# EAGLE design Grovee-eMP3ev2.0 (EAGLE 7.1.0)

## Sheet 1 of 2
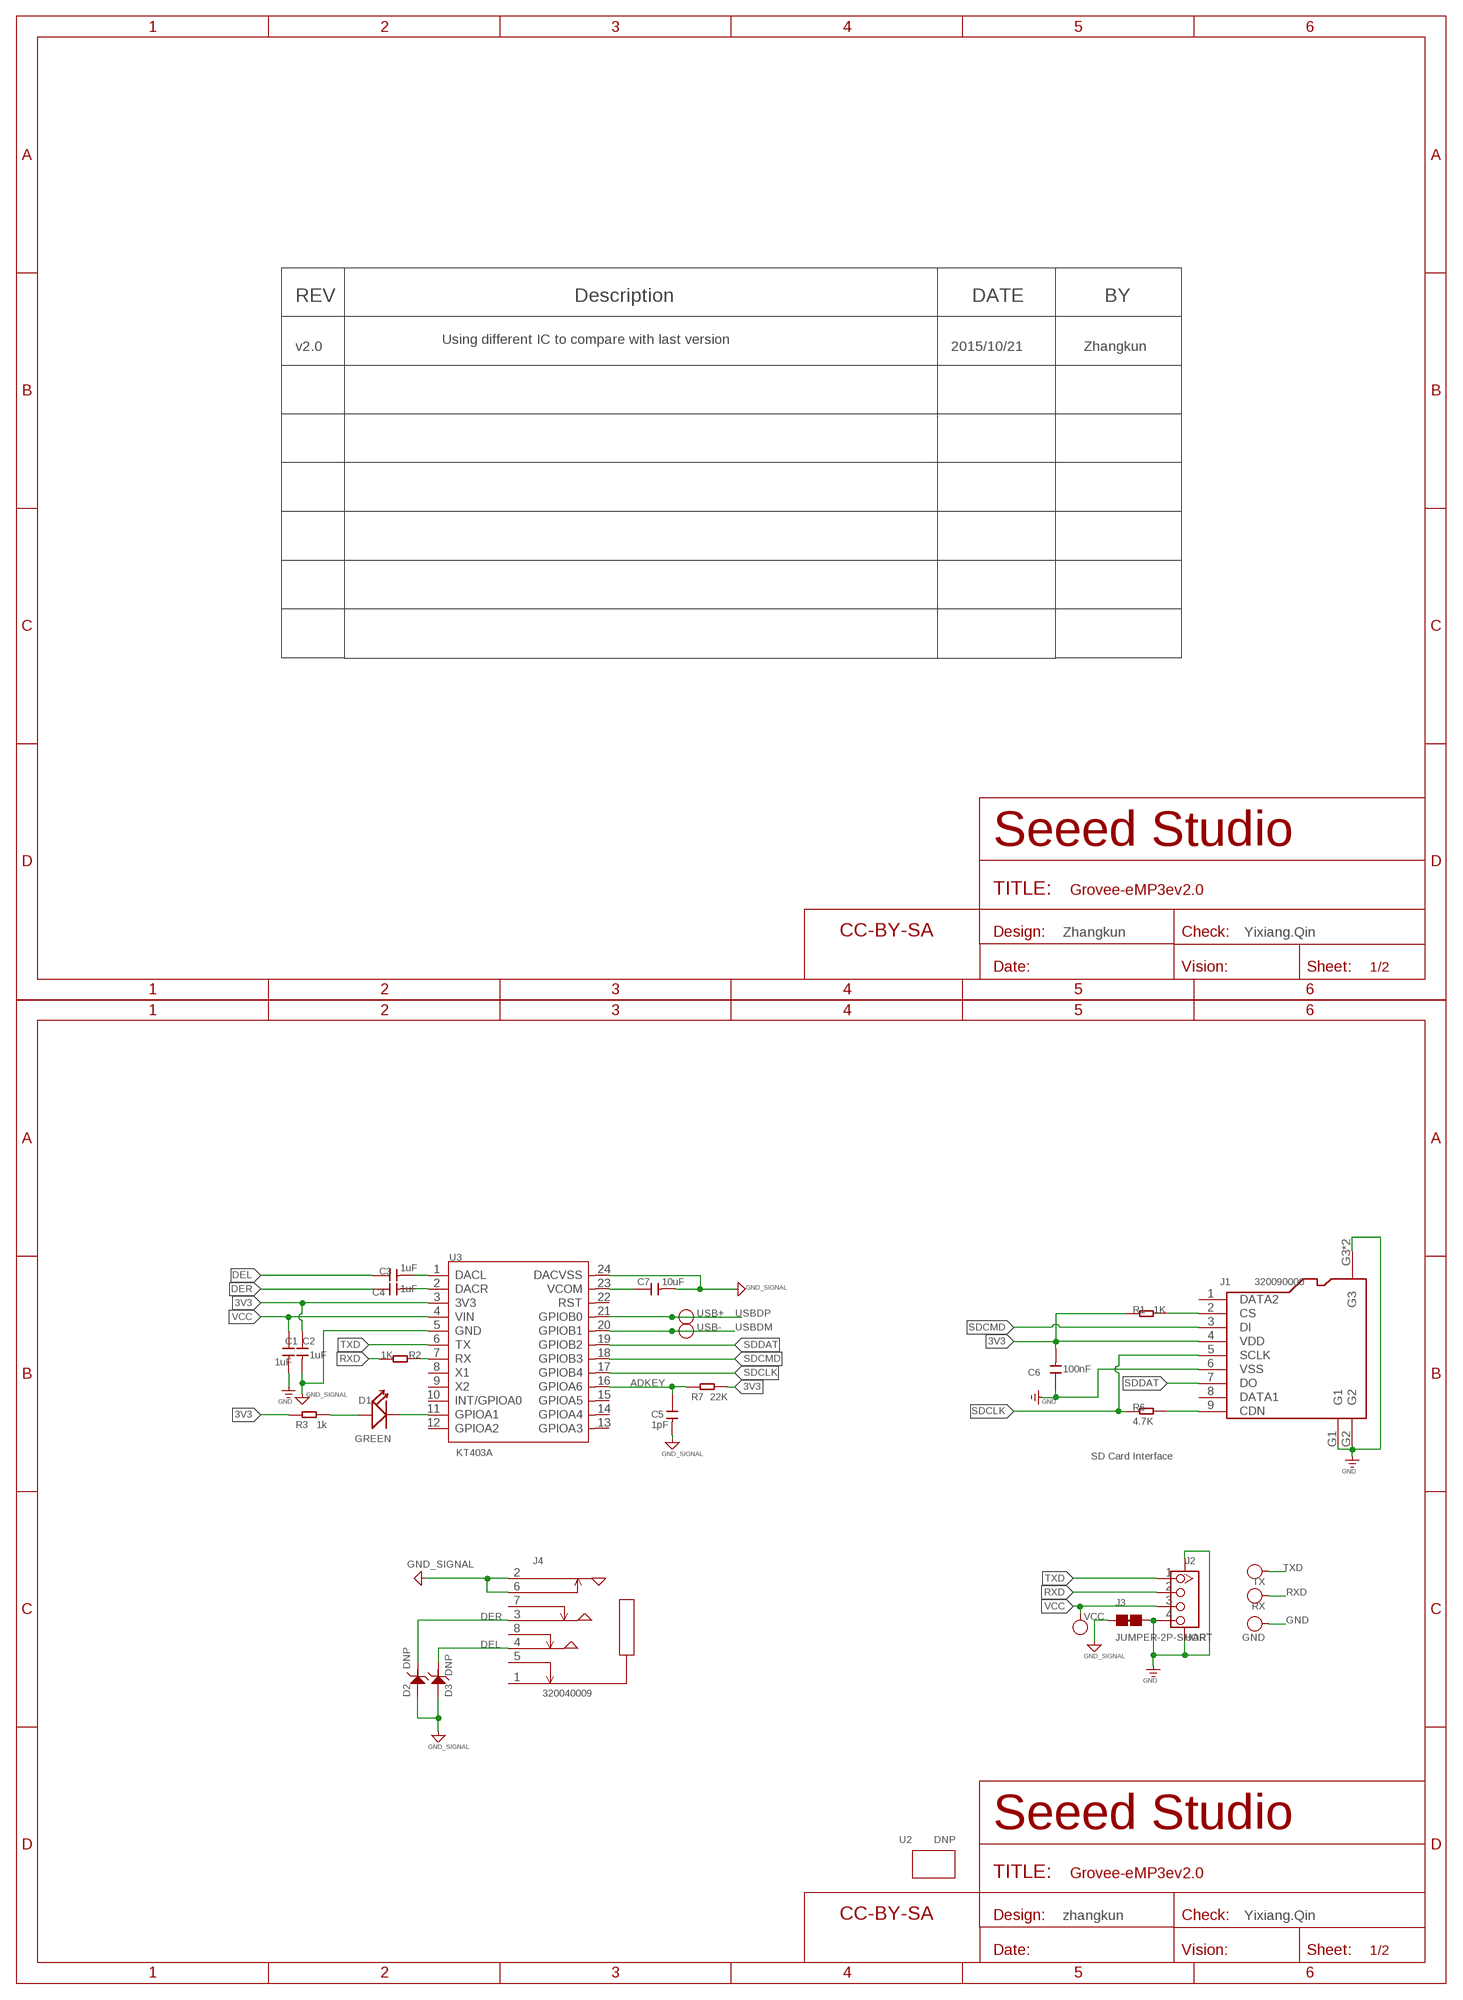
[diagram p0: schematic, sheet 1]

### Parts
C1  1uF  CAP-0402  [C0402]
C2  1uF  CAP-0402  [C0402]
C3  1uF  CAP-0402  [C0402]
C4  1uF  CAP-0402  [C0402]
C5  1pF  CAP-0402  [C0402]
C6  100nF  CAP-0402  [C0402]
C7  10uF  CAP-0402  [C0402]
D1  GREEN  LED'0603'  [LED-0603]
D2  DNP  D-ESD-2P'DF2S6.8FS'  [SOD-923]
D3  DNP  D-ESD-2P'DF2S6.8FS'  [SOD-923]
FR1  DNP  SEEEDSTUDIO-OPEN-SCH-FRAME  [SEEEDSTUDIO-PCB-FRAME]
FR2  DNP  SEEEDSTUDIO-OPEN-SCH-FRAME  [SEEEDSTUDIO-PCB-FRAME]
GND  DNP  TEST-POINT'4545'  [TP-D45MIL]
J1  320090000  MICRO-SD-CARD-HOLDER-9P'MICROSD-9P'  [MICRO-SD9+4P-SMD-16.1X14.5X1.85MM]
J2  UART  GROVE-CONNECTOR-SMD'DD'  [HW4-SMD-2.0]
J3  JUMPER-2P-SHORT  [2P-SMD-SHORT]
J4  320040009  AUDIO-JACK-8P-SMD'PJ-393'  [AUDIO8P-SMD-3.5-14.5X6.1X4.0MM]
R1  1K  RES-0402  [R0402]
R2  1K  R-0402  [R0402@1]
R3  1k  RES-0402  [R0402]
R6  4.7K  RES-0402  [R0402]
R7  22K  RES-0402  [R0402]
RX  DNP  TEST-POINT'4545'  [TP-D45MIL]
TX  DNP  TEST-POINT'4545'  [TP-D45MIL]
U2  DNP  GROVE'2U'  [GROVE-1*2-TEST-PLATFORM]
U3  KT403A  MCU-KT403A  [SSOP24-0.65-8.3X5.6MM]
USB+  DNP  TEST-POINT'4545'  [TP-D45MIL]
USB-  DNP  TEST-POINT'4545'  [TP-D45MIL]
VCC  DNP  TEST-POINT'4545'  [TP-D45MIL]

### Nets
3V3: C2.1 C6.2 J1.4(VDD) R1.2 R3.1 R7.2 U3.3(3V3)
ADKEY: C5.1 R7.1 U3.16(GPIOA6)
AGND: C2.2 C5.2 C7.2 D2.2 D3.2 J3.1 J4.2 J4.6 U3.5(GND) U3.24(DACVSS) ; supply symbol labelled GND_SIGNAL
DACR: C4.2 U3.2(DACR)
DEL: C3.1 D3.1 J4.4
DER: C4.1 D2.1 J4.3
GND: C1.2 C6.1 GND.T J1.6(VSS) J1.G1 J1.G2 J1.G3 J1.G4(G3) J2.4 J2.SS1 J2.SS2 J3.2
LD1: D1.- U3.11(GPIOA1)
N$1: D1.+ R3.2
N$2: C7.1 U3.23(VCOM)
N$3: J1.2(CS) R1.1
N$4: C3.2 U3.1(DACL)
N$8: J1.9(CDN) R6.1
RX_L: R2.1 U3.7(RX)
RXD: J2.2 R2.2 RX.T
SDCLK: J1.5(SCLK) R6.2 U3.17(GPIOB4)
SDCMD: J1.3(DI) U3.18(GPIOB3)
SDDAT: J1.7(DO) U3.19(GPIOB2)
TXD: J2.1 TX.T U3.6(TX)
USBDM: U3.20(GPIOB1) USB-.T
USBDP: U3.21(GPIOB0) USB+.T
VCC: C1.1 J2.3 U3.4(VIN) VCC.T
Unconnected: J1.1(DATA2) J1.8(DATA1) J4.1 J4.5 J4.7 J4.8 U3.8(X1) U3.9(X2) U3.10(INT/GPIOA0) U3.12(GPIOA2) U3.13(GPIOA3) U3.14(GPIOA4) U3.15(GPIOA5) U3.22(RST)

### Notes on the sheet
- REV | Description | DATE | BY
- Using different IC to compare with last version
- v2.0 | 2015/10/21 | Zhangkun
- Zhangkun | Yixiang.Qin
- SD Card Interface
- zhangkun | Yixiang.Qin

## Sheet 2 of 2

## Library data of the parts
C1-C7 = Discrete-new:CAP: Ceramic Capacitors
D1 = Discrete:LED*
D2 D3 = Discrete-new:D-ESD-2P: SOD-923:304060009;SOD-123:304060001
FR1 FR2 = moudle-new:SEEEDSTUDIO-OPEN-SCH-FRAME
GND RX TX USB+ USB- VCC = Discrete-new:TEST-POINT; PARTNO: DNP
J1 = Connector-new:MICRO-SD-CARD-HOLDER-9P: 320090000; SKU: 320090000
J2 = Connector-new:GROVE-CONNECTOR-SMD: 4P-SMD-2.0:320110030;4P-SMD-2.0-90D:320110032
J3 = Discrete-new:JUMPER-2P-SHORT
J4 = Connector-new:AUDIO-JACK-8P-SMD: 320040009
R1 R3 R6 R7 = Discrete-new:RES
R2 = Discrete:R*
U2 = moudle-new:GROVE
U3 = template:MCU-KT403A

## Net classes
0 default: width 0.203 mm, drill 0.305 mm, clearance 0.152 mm

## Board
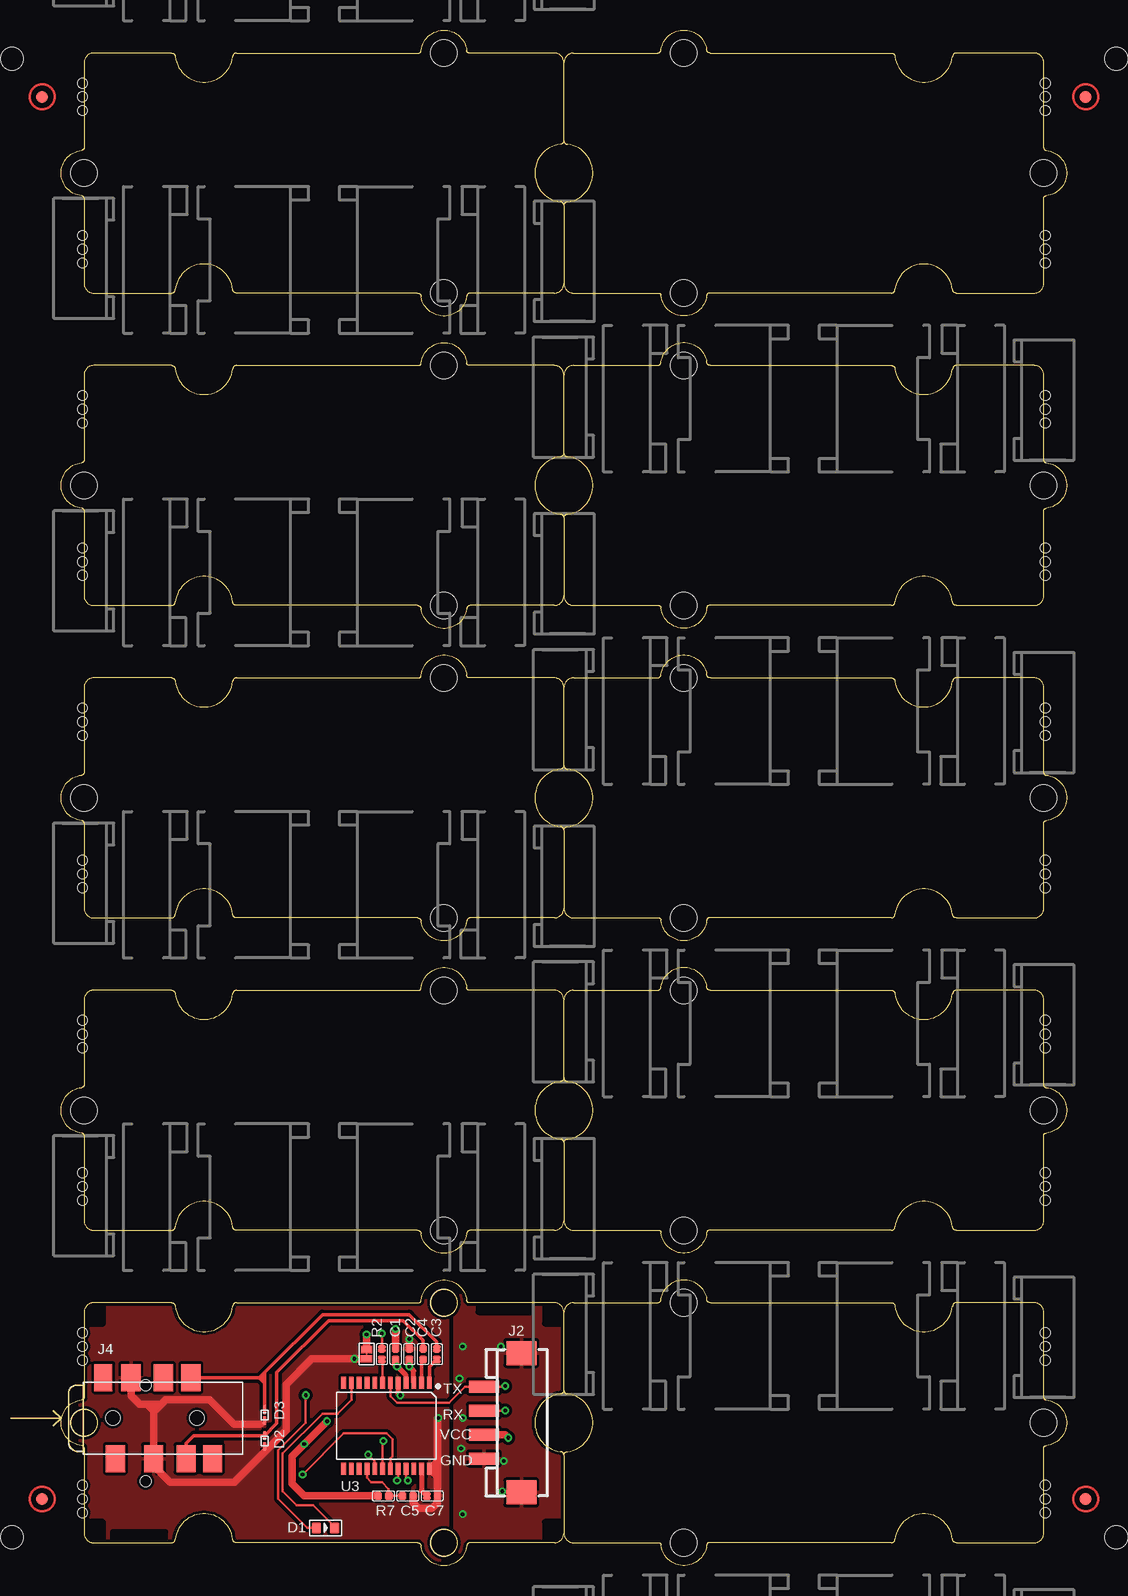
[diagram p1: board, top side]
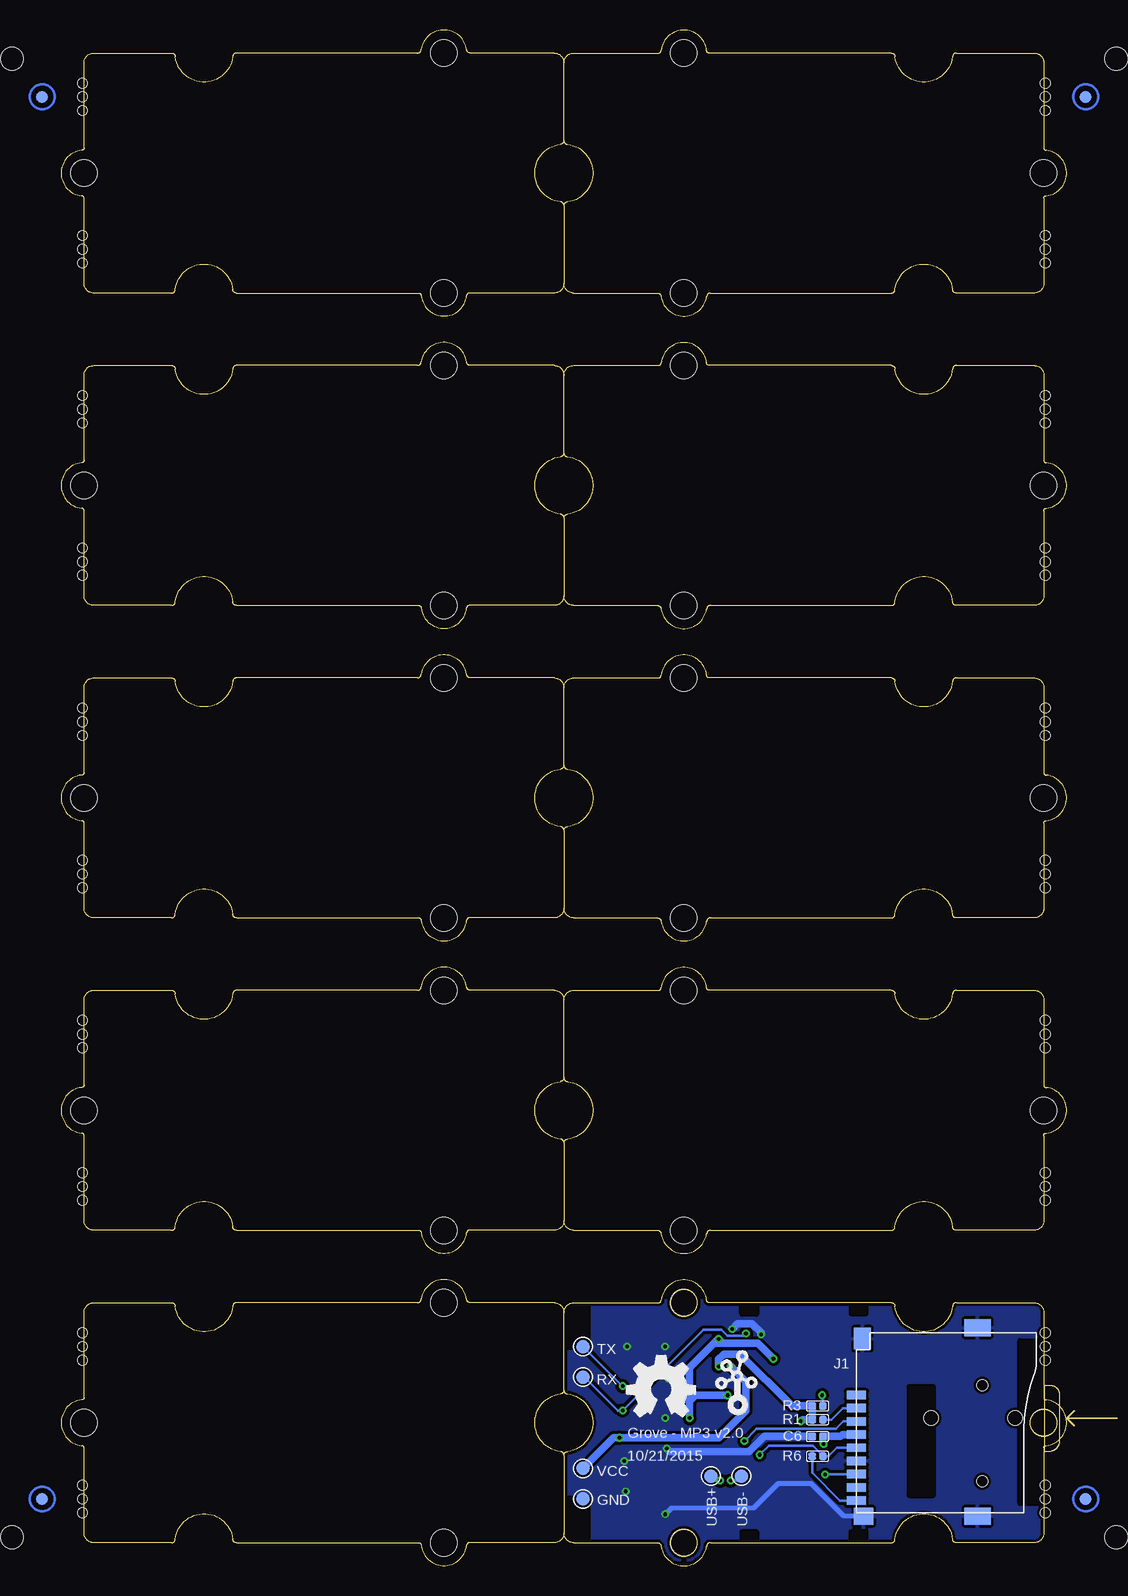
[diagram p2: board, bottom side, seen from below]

Size 83.82 x 127.98 mm. Coordinates in mm from the lower left corner, seen from the top.
Copper layers (1*16): Top 0.035mm / dielectric 1.5mm / Bottom 0.035mm
Design rules "SeeedStudio_2layer_DRU_no_angle_20140221 *": minimum track width 6mil, minimum drill 12mil, track to track 6mil, track to pad 6mil, pad to pad 6mil, via to via 6mil, smd to smd 0mil, copper to edge 10mil, drill to drill 10mil, minimum pad ring 10mil, minimum via ring 6mil, stop-mask expansion 2mil, vias tented up to drill 25mil, thermal gap 10mil
Holes 0.8 mm at 82.04,4.43 82.04,6.71 82.04,5.57 82.04,17.13 82.04,19.41 82.04,18.27 82.04,30.46 82.04,32.75 82.04,31.61 82.04,43.16 82.04,45.45 82.04,44.31 82.04,56.5 82.04,58.78 82.04,57.64 82.04,69.2 82.04,71.48 82.04,70.34 82.04,82.53 82.04,84.82 82.04,83.68 82.04,95.23 82.04,97.52 82.04,96.38 82.04,108.57 82.04,110.85 82.04,109.71 82.04,121.27 82.04,123.55 82.04,122.41 1.78,6.71 1.78,4.43 1.78,5.57 1.78,19.41 1.78,17.13 1.78,18.27 1.78,32.75 1.78,30.46 1.78,31.61 1.78,45.45 1.78,43.16 1.78,44.31 1.78,58.78 1.78,56.5 1.78,57.64 1.78,71.48 1.78,69.2 1.78,70.34 1.78,84.82 1.78,82.53 1.78,83.68 1.78,97.52 1.78,95.23 1.78,96.38 1.78,110.85 1.78,108.57 1.78,109.71 1.78,123.55 1.78,121.27 1.78,122.41
Holes 1.91 mm at 87.95,125.59 -4.13,125.59 -4.13,2.4 87.95,2.4

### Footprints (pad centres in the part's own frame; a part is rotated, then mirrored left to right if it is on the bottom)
C0402 = smd 0.635 x 0.635: 1 0,0.445; 2 0,-0.445
LED-0603 = smd 0.762 x 0.889: + -0.762,0; - 0.762,0
SOD-923 = smd 0.7 x 0.3: 1 -0.45,0; 2 0.45,0
TP-D45MIL = smd 1.143 x 1.143: T 0,0
MICRO-SD9+4P-SMD-16.1X14.5X1.85MM = smd 1.6 x 0.7: 1 0,2.25; 2 0,1.15; 3 0,0.05; 4 0,-1.05; 5 0,-2.15; 6 0,-3.25; 7 0,-4.35; 8 0,-5.45; 9 0,-6.55 | smd 1.6 x 1.4: G1 0.6,-7.85 | smd 2.2 x 1.4: G2 10.1,-7.85; G3 10.1,7.85 | smd 1.4 x 1.8: G4 0.5,6.95 | hole 0.9: 10.5,-4.95; 10.5,3.05
HW4-SMD-2.0 = smd 1 x 2.5: 1 -3,0; 2 -1,0; 3 1,0; 4 3,0 | smd 2 x 2.5: SS1 -5.8,3.123; SS2 5.8,3.123
2P-SMD-SHORT = smd 0.889 x 0.61: 1 0,0.381; 2 0,-0.381
AUDIO8P-SMD-3.5-14.5X6.1X4.0MM = smd 1.6 x 2.25: 1 3.9,-3.375; 2 7.1,-3.375; 3 9.8,-3.375; 4 10.2,3.375; 6 5.2,3.375; 7 7.9,3.375; 8 12,-3.375 | smd 1.5 x 2.25: 5 2.9,3.375 | hole 1.2: 3.7,0; 10.7,0
ROUND-MARK-1.0 = smd 1.016 x 1.016: P$1 0,0
R0402 = smd 0.635 x 0.635: 1 0,0.445; 2 0,-0.445
R0402@1 = smd 0.635 x 0.635: 1 -0.445,0; 2 0.445,0
GROVE-TEST-PLATFORM = hole 2.2: -10,-10; -10,10; 20,0
GROVE-1*2-TEST-PLATFORM = hole 2.2: 10.635,10; 10.635,-10; -19.365,0
SSOP24-0.65-8.3X5.6MM = smd 0.4 x 1: 1 -3.575,-3.6; 2 -2.925,-3.6; 3 -2.275,-3.6; 4 -1.625,-3.6; 5 -0.975,-3.6; 6 -0.325,-3.6; 7 0.325,-3.6; 8 0.975,-3.6; 9 1.625,-3.6; 10 2.275,-3.6; 11 2.925,-3.6; 12 3.575,-3.6; 13 3.575,3.6; 14 2.925,3.6; 15 2.275,3.6; 16 1.625,3.6; 17 0.975,3.6; 18 0.325,3.6; 19 -0.325,3.6; 20 -0.975,3.6; 21 -1.625,3.6; 22 -2.275,3.6; 23 -2.925,3.6; 24 -3.575,3.6

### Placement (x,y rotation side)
C1  27.88,17.64 180 top
C2  29.02,17.64 180 top
C3  31.31,17.64 0 top
C4  30.16,17.64 0 top
C5  28.89,5.83 90 top
C6  20.77,10.78 90 bottom
C7  30.93,5.83 90 top
D1  22.04,3.16 0 top
D2  16.96,10.4 270 top
D3  16.96,12.56 270 top
FR1  not placed on the board
FR2  not placed on the board
GND  40.32,5.57 0 bottom
J1  17.53,11.98 0 bottom
J2  35.24,11.92 270 top
J3  25.46,17.64 180 top
J4  0.62,12.3 0 top
P1  [ROUND-MARK-1.0]  85.41,122.41 180 top
P2  [ROUND-MARK-1.0]  -1.59,122.41 180 top
P3  [ROUND-MARK-1.0]  85.41,5.57 180 top
P4  [ROUND-MARK-1.0]  -1.59,5.57 180 top
P5  [ROUND-MARK-1.0]  85.41,122.41 180 bottom
P6  [ROUND-MARK-1.0]  -1.59,122.41 180 bottom
P7  [ROUND-MARK-1.0]  -1.59,5.57 180 bottom
P8  [ROUND-MARK-1.0]  85.41,5.57 180 bottom
R1  20.77,12.18 270 bottom
R2  26.73,17.64 90 top
R3  20.77,13.32 90 bottom
R6  20.77,9.13 90 bottom
R7  26.86,5.83 270 top
RX  40.32,15.73 0 bottom
TX  40.32,18.27 0 bottom
U1  [GROVE-TEST-PLATFORM]  21.91,90.03 180 top
U2  21.27,11.92 0 top
U3  27.12,11.67 180 top
U4  [GROVE-TEST-PLATFORM]  61.91,90.03 0 top
U5  [GROVE-TEST-PLATFORM]  21.91,63.99 180 top
U6  [GROVE-TEST-PLATFORM]  61.91,63.99 0 top
U7  [GROVE-TEST-PLATFORM]  21.91,37.96 180 top
U8  [GROVE-TEST-PLATFORM]  61.91,37.96 0 top
U9  [GROVE-TEST-PLATFORM]  61.91,11.92 0 top
U10  [GROVE-TEST-PLATFORM]  21.91,11.92 180 top
U11  [GROVE-TEST-PLATFORM]  21.91,116.06 180 top
U12  [GROVE-TEST-PLATFORM]  61.91,116.06 0 top
U$7  [OSHW_FILLX200_NOTEXT]  36.64,12.43 0 bottom
U$10  [GROVE-SILK-SMALL]  29.66,12.43 0 bottom
USB+  29.66,7.48 90 bottom
USB-  27.12,7.48 90 bottom
VCC  40.32,8.11 0 bottom

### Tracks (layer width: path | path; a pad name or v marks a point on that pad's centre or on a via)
3V3  (via drill 0.3 pad 0.64)
  Top 0.406: U3.3 29.39,16.25 v29.02,16.62
  Top 0.61: C2.1 v29.02,16.62 | R7.2 20.26,5.83 19.24,6.84 19.24,9.13 v20.26,10.14 v22.16,12.05
  Bottom 0.61: v29.02,16.62 C2.1 28.58,17.64 27.24,17.64 22.92,13.32 R3.1 R1.2 22.04,12.18 v22.16,12.05 | v20.26,10.14 20.32,10.21 C6.2 18.86,10.78 18.7,10.94 J1.4
ADKEY
  Top 0.203: U3.16 25.49,7.32 25.85,6.97 26.73,6.97 27.31,6.4 R7.1 C5.1
AGND  (via drill 0.3 pad 0.64)
  Top 0.305: D3.2 16.96,11.92 16.83,11.79 16.57,11.79 | 16.96,9.51 D2.2
  Top 0.406: U3.5 28.09,14.38 v28.26,14.21 | U3.24 31.33,8.07 31.37,8.11 | U3.24 30.69,8.13 31.31,8.75 | U3.24 30.69,7.97 31.31,7.35
  Top 0.61: C2.2 v29.02,18.91 | C5.2 29.34,5.25 29.78,4.81 30.93,4.81 31.37,5.25 C7.2 31.37,8.11 31.37,12.24 v31.43,12.3 | 16.57,11.79 14.42,11.79 12.38,13.83 8.7,13.83 8.32,13.45 | 8.32,13.45 7.68,13.45 | 7.68,13.45 7.18,13.45 | 7.18,13.45 6.54,13.45 5.82,14.17 J4.6 | 7.72,12.84 J4.2 7.72,8.33 9.08,6.97 14.42,6.97 16.96,9.51 18.73,11.29 18.73,15.1 20.89,17.26 v24.45,17.26 J3.1 | 7.72,12.91 7.72,13.41 7.68,13.45 | 7.72,12.84 7.72,12.91 | 7.72,12.91 7.18,13.45 | 7.72,12.84 8.32,13.45
  Bottom 0.61: v31.43,12.3 31.43,13.7 | 31.43,13.7 31.43,14.21 | 31.43,14.21 31.43,14.72 | 31.43,14.72 31.43,16.49 29.4,18.53 | 29.4,18.53 v29.02,18.91 28.64,18.53 | v28.26,14.21 30.93,14.21 | 30.93,14.21 31.43,14.21 | 30.93,14.21 31.43,14.72 | 30.93,14.21 31.43,13.7 | 28.64,18.53 25.72,18.53 v24.45,17.26 | 28.64,18.53 29.4,18.53
  pour Top (isolate 0.254): 1.59,22.08 32.2,22.08 32.2,0.49 1.59,0.49
DACR
  Top 0.305: U3.2 30.04,17.07 C4.2
DEL
  Top 0.305: J4.4 16.5,15.68 | 16.52,15.68 16.9,15.68 16.96,15.73 | 16.96,16.11 21.78,20.94 29.02,20.94 31.31,18.65 C3.1 31.31,18.02 | D3.1 16.96,15.22 | 16.96,15.22 16.96,15.73 | 16.96,15.73 16.96,16.11 | 16.5,15.68 16.52,15.68 | 16.52,15.68 16.96,16.11 | 16.5,15.68 16.96,15.22
DER
  Top 0.305: J4.3 10.42,10.21 11.06,10.85 D2.1 17.97,11.86 17.97,16.11 22.29,20.43 28.51,20.43 30.16,18.78 C4.1
GND  (via drill 0.3 pad 0.64)
  Top 0.61: C1.2 v27.88,19.73 | J3.2 v25.46,19.29
  Bottom 0.406: J1.G1 18.57,4.13 21.27,6.84 24.07,6.84 26.1,4.81 32.96,4.81 v33.47,4.3
  Bottom 0.61: v25.46,19.29 25.46,19.41 26.23,20.18 27.43,20.18 v27.88,19.73 | C6.1 25.21,10.78 26.48,9.51 33.08,9.51 v33.34,9.76
  other vias: 36.89,8.75 33.21,15.6 33.47,12.3 33.47,18.27 36.64,18.27 36.77,6.21
  pour Bottom (isolate 0.254): 1.59,22.08 42.36,22.08 42.36,0.49 1.59,0.49
  pour Top (isolate 0.254): 32.83,22.72 42.36,22.72 42.36,1.13 32.83,1.13
LD1
  Top 0.203: D1.- 22.8,3.26 20.99,5.06 19.62,5.06 18.48,6.21 18.48,9.38 21.78,12.68 23.05,12.68 24.19,13.82 U3.11
N$1  (via drill 0.3 pad 0.64)
  Top 0.203: v20.38,14.21 20.38,11.92 18.1,9.64 18.1,5.57 20.51,3.16 D1.+
  Bottom 0.203: R3.2 20.32,14.14 v20.38,14.21
N$2
  Top 0.406: U3.23 30.04,6.27 C7.1
N$3
  Bottom 0.203: R1.1 19.62,12.18 18.66,13.13 J1.2
N$4
  Top 0.305: U3.1 30.69,16.58 C3.2
N$8
  Bottom 0.203: J1.9 18.9,5.44 21.21,7.74 R6.1
RX_L
  Top 0.203: U3.7 26.79,17.14 R2.1
RXD  (via drill 0.3 pad 0.64)
  Top 0.203: R2.2 v26.73,19.35 | J2.2 37.01,12.92 v37.02,12.94
  Bottom 0.203: RX.T 40.21,15.73 37.42,12.94 v37.02,12.94 30.29,19.67 28.77,19.67 28.26,19.16 26.86,19.16 26.73,19.29 v26.73,19.35
SDCLK  (via drill 0.3 pad 0.64)
  Top 0.203: U3.17 26.14,8.71 v25.59,9.25
  Bottom 0.203: J1.5 19.17,9.83 19.88,9.13 R6.2 20.32,9.19 21.15,10.02 24.83,10.02 v25.59,9.25
SDCMD  (via drill 0.3 pad 0.64)
  Top 0.203: U3.18 26.79,10.33 v26.86,10.4
  Bottom 0.203: J1.3 18.62,12.04 19.24,11.41 25.85,11.41 v26.86,10.4
SDDAT  (via drill 0.3 pad 0.64)
  Top 0.203: v20.13,7.6 23.56,11.03 27.12,11.03 27.62,10.52 27.62,9.13 27.44,8.94 U3.19
  Bottom 0.203: J1.7 20.1,7.63 v20.13,7.6
TXD  (via drill 0.3 pad 0.64)
  Top 0.203: U3.6 27.44,14.14 28,13.57 32.32,13.57 33.67,14.92 J2.1 36.97,14.92 v37.02,14.97
  Bottom 0.203: v37.02,14.97 TX.T
USBDM  (via drill 0.3 pad 0.64)
  Top 0.203: U3.20 28.09,7.18 v28,7.1
  Bottom 0.203: v28,7.1 27.5,7.1 USB-.T
USBDP  (via drill 0.3 pad 0.64)
  Top 0.203: v28.89,7.1 28.74,7.25 U3.21
  Bottom 0.203: v28.89,7.1 29.27,7.1 USB+.T
VCC  (via drill 0.3 pad 0.64)
  Top 0.406: U3.4 28.74,15.88 v28,16.62
  Top 0.61: C1.1 27.88,16.75 v28,16.62 | J2.3 37.02,10.92 v37.28,10.67
  Bottom 0.61: VCC.T 37.77,10.67 v37.28,10.67 29,10.67 26.73,12.94 26.73,15.35 v28,16.62

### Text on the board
tPlace: TX | RX | VCC | GND
bPlace: Grove - MP3 v2.0 | 10/21/2015

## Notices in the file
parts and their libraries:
moudle-new: This work is licensed under the Creative Commons Attribution 4.0 International License.
To view a copy of this license,visit:
http://creativecommons.org/licenses/by-sa/4.0
moudle-new: CC-BY-SA
